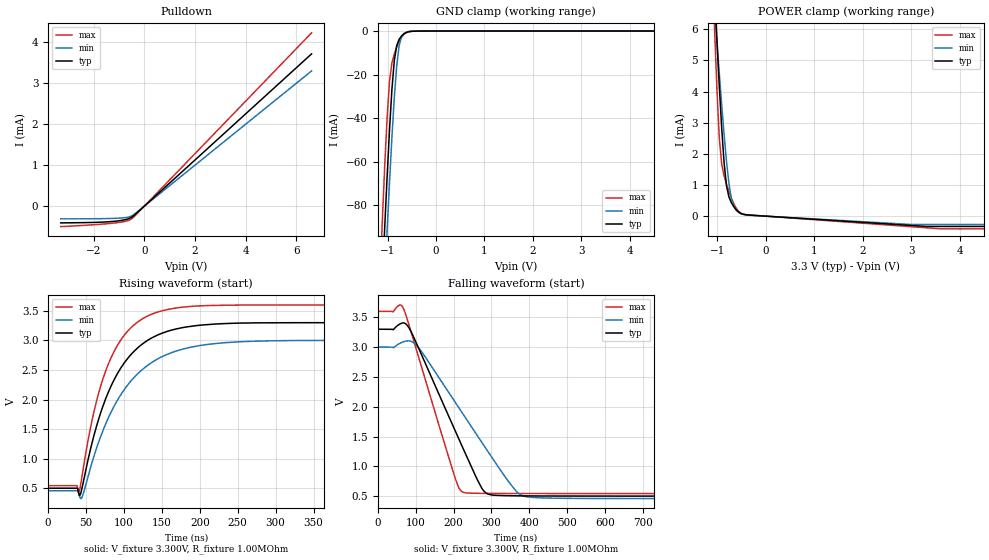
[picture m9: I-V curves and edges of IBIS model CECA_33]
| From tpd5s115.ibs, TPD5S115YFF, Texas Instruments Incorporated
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[Model]   CECA_33
Model_type   I/O_open_sink
Vinl = 0.2706V
Vinh = 2.31V
Vmeas = 1.6025V
Cref = 15pF
Vref = 0V
Rref = 1000000
|   typ   min   max
|3-state
C_comp   1.1344pF   1.1015pF   1.2192pF
|pulldown
|C_comp   1.1344pF   1.1015pF   1.2166pF
[Voltage Range]   3.300V   3.00V   3.6V
|Junction temperature
[Temperature Range]   40.0   100.0   -40.0
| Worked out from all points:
|   slope of the pulldown table from 0 to 0.495 V, typ, clamps not added: 1.78 kohm
|   GND clamp passes 1 mA (typ) near -0.64 V on its own axis
|   POWER clamp passes 1 mA (typ) near -0.81 V on its own axis
|   falling waveform, V_fixture 3.300V, R_fixture 1.00MOhm: 20-80 % time 118ns typ, 160ns min, 86.9ns max; typ from 3.3 V to 0.5 V
|   rising waveform, V_fixture 3.300V, R_fixture 1.00MOhm: 20-80 % time 53.8ns typ, 64.2ns min, 44.5ns max; typ from 0.5 V to 3.3 V
|ambient temperature   25   85   -40|
[Pulldown]
|   Voltage   I(typ)   I(min)   I(max)
-3.3V     -408uA     -310uA     -499uA
-1.26V    -374.2uA   -299.8uA   -416.6uA
-713.1mV  -323.4uA   -276.2uA   -364.4uA
-464.3mV  -254.2uA   -225.1uA   -290.7uA
6.6V      3.714mA    3.298mA    4.228mA
[GND Clamp]
|   Voltage   I(typ)   I(min)   I(max)
-3.3V     -2.285A    -2.051A    -2.629A
-1.161V   -140.4mA   -164mA     -114.1mA
-1.111V   -115.1mA   -139.3mA   -87.51mA
-1.061V   -90.52mA   -115.3mA   -62.41mA
-1.012V   -67.11mA   -91.95mA   -40mA
-961.8mV  -45.48mA   -69.67mA   -23.17mA
-912.1mV  -26.88mA   -48.92mA   -14.71mA
-862.3mV  -13.5mA    -30.52mA   -10.56mA
-812.6mV  -6.659mA   -15.92mA   -7.423mA
-713.1mV  -2.253mA   -2.629mA   -2.864mA
-613.6mV  -659.8uA   -538.9uA   -689.6uA
6.6V      0A         0A         0A
[POWER Clamp]
|   Voltage   I(typ)   I(min)   I(max)
-3.3V     65.62mA    7.928mA    101.1mA
-1.061V   7.235mA    6.729mA    6.104mA
-1.012V   5.665mA    5.643mA    4.086mA
-961.8mV  4.175mA    4.586mA    2.508mA
-912.1mV  2.82mA     3.569mA    1.665mA
-862.3mV  1.704mA    2.613mA    1.292mA
-812.6mV  972uA      1.753mA    1.026mA
-713.1mV  434.4uA    569.2uA    581.2uA
-613.6mV  207.3uA    190uA      257uA
-514.1mV  85.98uA    78.49uA    91.47uA
3.615V    -330uA     -268uA     -407.5uA
6.6V      -330uA     -268uA     -407.5uA
[Ramp]
R_load = 1.00MOhm
|   typ   min   max
dV/dt_r   1.680V/53.788ns   1.526V/64.202ns   1.834V/44.485ns
dV/dt_f   1.680V/117.748ns   1.526V/159.862ns   1.834V/86.888ns
[Falling Waveform]
V_fixture = 3.300V
V_fixture_min = 3.000V
V_fixture_max = 3.600V
R_fixture = 1.00MOhm
|   Time   V(typ)   V(min)   V(max)
0s        3.3V       3V         3.6V
40ns      3.29V      2.993V     3.591V
67ns      3.406V     3.089V     3.653V
106ns     3.005V     3.001V     2.862V
203ns     1.614V     2.088V     823.9mV
228ns     1.259V     1.848V     558.7mV
286ns     551.9mV    1.294V     545.7mV
366ns     504.9mV    578.6mV    543.7mV
397ns     503.3mV    485.2mV    543.4mV
1.9us     499.8mV    456.7mV    542.7mV
[Rising Waveform]
V_fixture = 3.300V
V_fixture_min = 3.000V
V_fixture_max = 3.600V
R_fixture = 1.00MOhm
|   Time   V(typ)   V(min)   V(max)
0s        499.8mV    456.7mV    542.7mV
38ns      499.8mV    456.7mV    542.7mV
41ns      378.6mV    396mV      445.2mV
45ns      519mV      357.8mV    728.2mV
64ns      1.557V     1.183V     1.984V
89ns      2.384V     1.935V     2.862V
122ns     2.917V     2.482V     3.346V
173ns     3.205V     2.836V     3.556V
323ns     3.299V     2.998V     3.6V
1.9us     3.3V       3V         3.6V
